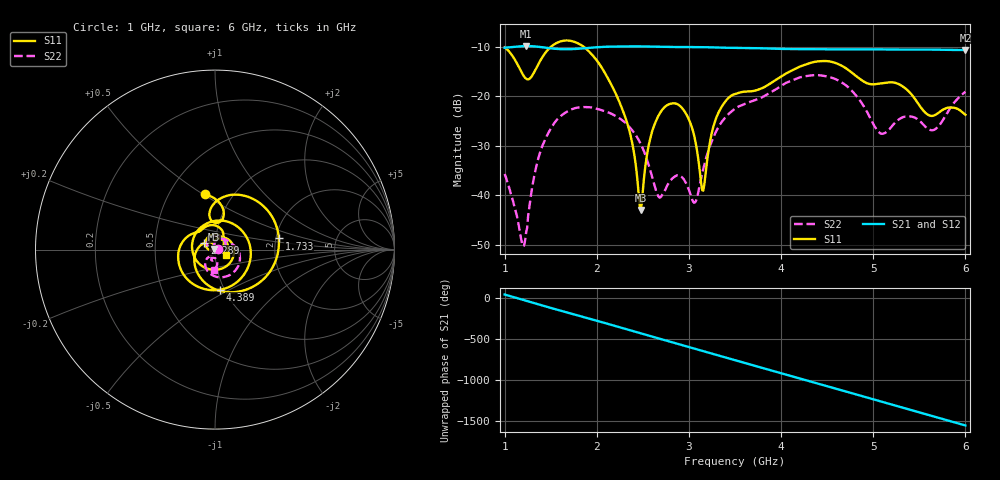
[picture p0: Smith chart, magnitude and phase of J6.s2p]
!Agilent Technologies,E8364B,MY43040528,A.07.50.67
!Agilent E8364B: A.07.50.67
!Date: Sunday, March 01, 2026 19:05:21
!Correction: S11(Full 2 Port(1,2))
!S21(Full 2 Port(1,2))
!S12(Full 2 Port(1,2))
!S22(Full 2 Port(1,2))
!S2P File: Measurements: S11, S21, S12, S22:
# Hz S  dB  R 50
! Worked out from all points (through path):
!   451 points, 1 GHz to 6 GHz, reference 50 ohm
!   highest |S21| = -9.82 dB at 1.233 GHz (marker M1); lowest = -10.6 dB at 6 GHz (marker M2)
!   group delay of S21, straight-line fit = 889 ps
!   lowest |S11| = -42.9 dB at 2.478 GHz (marker M3), VSWR 1.01, Z = 49.4 + j0.379 ohm
!   |S11| at or under -10 dB: start of sweep to 1.501 GHz; 1.86 GHz to end of sweep
!   |S22| runs from -50.2 to -15.7 dB; largest |S21 - S12| = 0.0014
!   S11 on the Smith chart (normalised r, x): 1 GHz: 0.74, +0.51; 1.733 GHz: 2.08, +0.30; 2.289 GHz: 0.89, +0.07; 4.389 GHz: 0.95, -0.45; 6 GHz: 1.12, -0.06
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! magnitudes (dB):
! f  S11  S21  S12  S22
! 1 GHz  -10.1  -10.2  -10.2  -35.6
! 1.189 GHz  -15.3  -9.8  -9.9  -49.6
! 1.233 GHz  -16.4  -9.8  -9.8  -47.5
! 1.4 GHz  -12.4  -10.1  -10.1  -30.5
! 1.733 GHz  -8.8  -10.4  -10.5  -22.6
! 1.844 GHz  -9.8  -10.3  -10.3  -22.2
! 2.289 GHz  -23.2  -9.9  -9.9  -25.0
! 2.389 GHz  -29.8  -9.9  -9.9  -26.9
! 2.478 GHz  -42.9  -9.9  -9.9  -29.6
! 2.567 GHz  -29.6  -9.9  -10.0  -34.0
! 2.667 GHz  -24.0  -10.0  -10.0  -40.1
! 2.956 GHz  -23.1  -10.0  -10.1  -37.1
! 3.067 GHz  -28.8  -10.0  -10.1  -41.4
! 3.156 GHz  -39.0  -10.1  -10.1  -34.6
! 3.289 GHz  -24.7  -10.1  -10.1  -27.3
! 3.5 GHz  -19.5  -10.2  -10.2  -22.5
! 4.344 GHz  -13.1  -10.5  -10.5  -15.7
! 4.389 GHz  -12.9  -10.5  -10.5  -15.7
! 5.167 GHz  -17.2  -10.5  -10.6  -26.8
! 5.378 GHz  -18.8  -10.5  -10.6  -24.0
! 5.667 GHz  -23.8  -10.6  -10.6  -26.7
! 6 GHz  -23.7  -10.6  -10.7  -19.0
